(* Logix 5000 AddOnInstructionDefinition export AMCI_SMD34E2_Axis_Follower_Linear; software revision 20.03 *)

ADD_ON_INSTRUCTION AMCI_SMD34E2_Axis_Follower_Linear   (* revision 1.0, vendor AMCI, ExecuteEnableInFalse *)
VAR_OUTPUT
   EN : BOOL; {visible}
END_VAR
VAR_INPUT
   Axis_Status_Bits : INT; {required}
   Follower_Type_Motor_or_Encoder : BOOL; {required}
   Follower_Position : REAL; {required}
   Follower_Velocity : REAL; {required}
   Acceleration : INT; {required}
   Deceleration : INT; {required}
   Proportional_Coefficient : INT; {required}
   Network_delay : INT; {required}
END_VAR
VAR_OUTPUT
   Axis_Follower_occurring : BOOL; {visible}
END_VAR
VAR_IN_OUT
   AMCI_SMD34E2_output_data : _000A:SMD34E2_788832CB:O:0; {required}
END_VAR
VAR_OUTPUT
   ER : BOOL; {visible}
END_VAR
VAR
   command_data_block : INT[10];
        [0]   // Command Bits MSW
        [1]   // Command Bits LSW
        [2]   // Upper Target Position
        [3]   // Lower Target Position
        [4]   // Upper Programmed Speed
        [5]   // Lower Programmed Speed
   axis_follower_position : DINT;
   axis_follower_velocity : DINT;
END_VAR

ROUTINE EnableInFalse   (* ladder *)
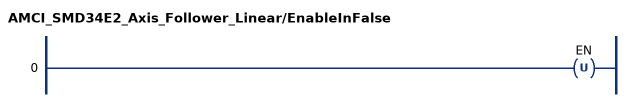
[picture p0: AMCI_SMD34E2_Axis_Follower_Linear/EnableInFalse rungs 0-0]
   0: OTU(EN);
END_ROUTINE

ROUTINE Logic   (* ladder *)
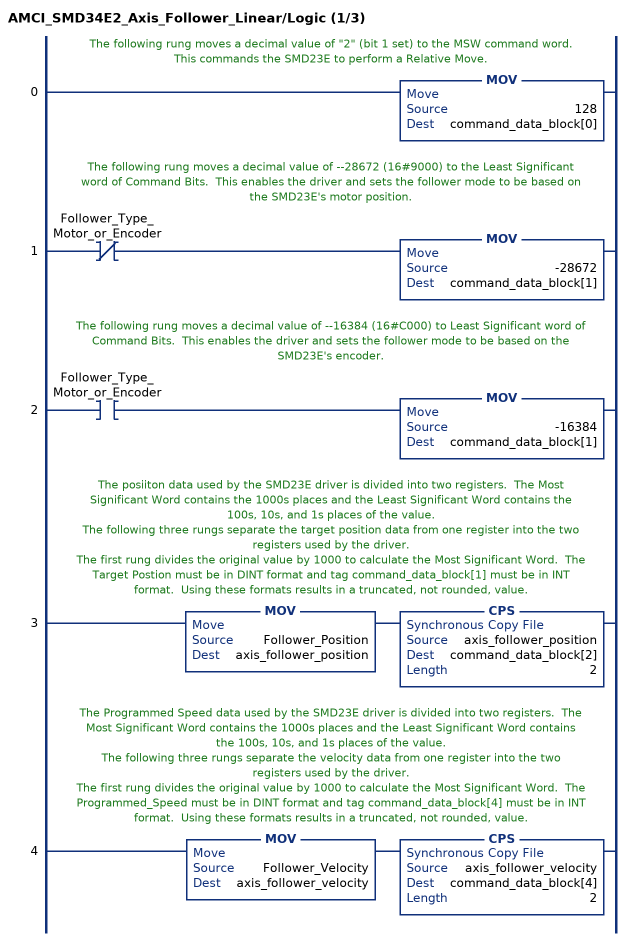
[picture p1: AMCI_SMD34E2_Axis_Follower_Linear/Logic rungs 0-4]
   // The following rung moves a decimal value of "2" (bit 1 set) to the MSW command word.  This commands the SMD23E to perform a Relative Move.
   0: MOV(128,command_data_block[0]);
   // The following rung moves a decimal value of --28672 (16#9000) to the Least Significant word of Command Bits.  This enables the driver and sets the follower mode to be based on the SMD23E's motor position.
   1: XIO(Follower_Type_Motor_or_Encoder)MOV(-28672,command_data_block[1]);
   // The following rung moves a decimal value of --16384 (16#C000) to Least Significant word of Command Bits.  This enables the driver and sets the follower mode to be based on the SMD23E's encoder.
   2: XIC(Follower_Type_Motor_or_Encoder)MOV(-16384,command_data_block[1]);
   // The posiiton data used by the SMD23E driver is divided into two registers.  The Most Significant Word contains the 1000s places and the Least Significant Word contains the 100s, 10s, and 1s places of the value.
   // The following three rungs separate the target position data from one register into the two registers used by the driver.
   // The first rung divides the original value by 1000 to calculate the Most Significant Word.  The Target Postion must be in DINT format and tag command_data_block[1] must be in INT format.  Using these formats results in a truncated, not rounded, value.
   3: MOV(Follower_Position,axis_follower_position)CPS(axis_follower_position,command_data_block[2],2);
   // The Programmed Speed data used by the SMD23E driver is divided into two registers.  The Most Significant Word contains the 1000s places and the Least Significant Word contains the 100s, 10s, and 1s places of the value.
   // The following three rungs separate the velocity data from one register into the two registers used by the driver.
   // The first rung divides the original value by 1000 to calculate the Most Significant Word.  The Programmed_Speed must be in DINT format and tag command_data_block[4] must be in INT format.  Using these formats results in a truncated, not rounded, value.
   4: MOV(Follower_Velocity,axis_follower_velocity)CPS(axis_follower_velocity,command_data_block[4],2);
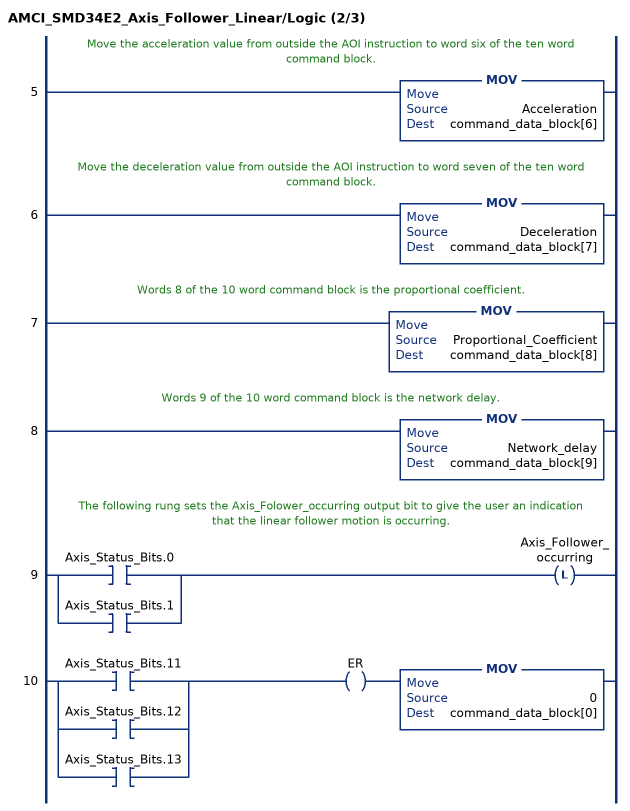
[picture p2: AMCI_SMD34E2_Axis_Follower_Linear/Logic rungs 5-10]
   // Move the acceleration value from outside the AOI instruction to word six of the ten word command block.
   5: MOV(Acceleration,command_data_block[6]);
   // Move the deceleration value from outside the AOI instruction to word seven of the ten word command block.
   6: MOV(Deceleration,command_data_block[7]);
   // Words 8 of the 10 word command block is the proportional coefficient.
   7: MOV(Proportional_Coefficient,command_data_block[8]);
   // Words 9 of the 10 word command block is the network delay.
   8: MOV(Network_delay,command_data_block[9]);
   // The following rung sets the Axis_Folower_occurring output bit to give the user an indication that the linear follower motion is occurring.
   9: [XIC(Axis_Status_Bits.0) ,XIC(Axis_Status_Bits.1) ]OTL(Axis_Follower_occurring);
   10: [XIC(Axis_Status_Bits.11) ,XIC(Axis_Status_Bits.12) ,XIC(Axis_Status_Bits.13) ]OTE(ER)MOV(0,command_data_block[0]);
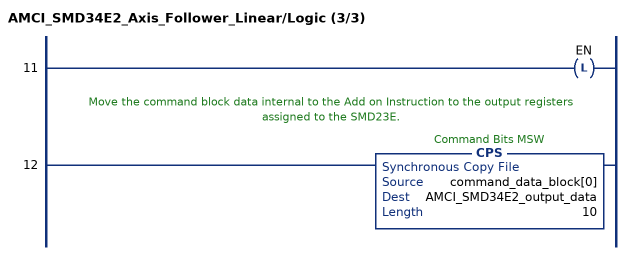
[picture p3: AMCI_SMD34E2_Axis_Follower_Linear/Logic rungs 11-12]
   11: OTL(EN);
   // Move the command block data internal to the Add on Instruction to the output registers assigned to the SMD23E.
   12: CPS(command_data_block[0],AMCI_SMD34E2_output_data,10);
END_ROUTINE
END_ADD_ON_INSTRUCTION
